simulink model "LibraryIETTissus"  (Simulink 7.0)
settings: Solver=ode45  StartTime=0.0  StopTime=10  RelTol=1e-3
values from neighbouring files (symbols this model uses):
  b = S/Sm    (= 0.1)    [Constantes.m]    (also in ConstantesBck.m)
  beta = 0.95    [Constantes.m]    (also in ResCourV1.m = 1; ResCrV1.m = 1; ResEnerV1.m = 1; ConstantesBck.m)
  C = 1    [Constantes.m]    (also in ConstantesBck.m)
  Cdl = 603E-9    (= 6.03e-07)    [Constantes.m]    (also in ResCourV1.m = 7.313e-07; ResCrV1.m = 7.313e-07; ResEnerV1.m = 7.313e-07; ConstantesBck.m)
  Cmem = 1E-6*Sm*(1-b)    (= 2.826e-08)    [Constantes.m]    (also in ConstantesBck.m = 3.14e-11; ImpedanceZtissus.m = 4e-08; Ztissus.m = 4e-08; CalculCharge.m = 1)
  Fact = 10^2    (= 100)    [Constantes.m]    (also in ConstantesBck.m)
  gk = 36    [Constantes.m]    (also in ConstantesBck.m; sim_hh.m)
  gl = 0.3    [Constantes.m]    (also in ConstantesBck.m; sim_hh.m)
  gna = 120    [Constantes.m]    (also in ConstantesBck.m; sim_hh.m)
  h0 = 0.5961    [Constantes.m]    (also in ConstantesBck.m)
  m0 = 0.0529    [Constantes.m]    (also in ConstantesBck.m)
  mK = 0    [Constantes.m]    (also in ConstantesBck.m)
  mL = 0    [Constantes.m]    (also in ConstantesBck.m)
  mNa = 0    [Constantes.m]    (also in ConstantesBck.m)
  n0 = 0.3177    [Constantes.m]    (also in ConstantesBck.m)
  rapportIE = 10    [Constantes.m]
  Rcan = 6.398E3*Sm*(1-b)    (= 180.80748)    [Constantes.m]    (also in ConstantesBck.m = 0.03454; ImpedanceZtissus.m = 44; Ztissus.m = 44)
  Rct = 185.6E3    (= 185600)    [Constantes.m]    (also in ResCourV1.m = 605200; ResCrV1.m = 605200; ResEnerV1.m = 605200; ConstantesBck.m)
  Rext = 2.9E3    (= 2900)    [Constantes.m]    (also in ConstantesBck.m)
  Rint = 2.9E2    (= 290)    [Constantes.m]    (also in ConstantesBck.m = 400)
  sigma = 66466    [Constantes.m]    (also in ResCourV1.m = 68000; ResCrV1.m = 68000; ResEnerV1.m = 68000; ConstantesBck.m)
  Sm = 3.14e-2    (= 0.0314)    [Constantes.m]    (also in ConstantesBck.m = 0.000314)
  Vk = -82    [Constantes.m]    (also in ConstantesBck.m)
  Vl = -59    [Constantes.m]    (also in ConstantesBck.m)
  Vna = 45    [Constantes.m]    (also in ConstantesBck.m)
  Vr = -70    [Constantes.m]    (also in ConstantesBck.m)
undefined symbols (not defined in the file or in its folder): ln
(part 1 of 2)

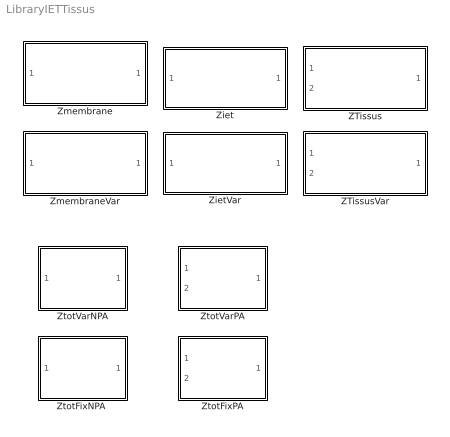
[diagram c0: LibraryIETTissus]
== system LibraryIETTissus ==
  ZTissus : Subsystem
  ZTissusVar : Subsystem
  Ziet : Subsystem
  ZietVar : Subsystem
  Zmembrane : Subsystem
  ZmembraneVar : Subsystem
  "ZtotFixNPA " : Subsystem
  ZtotFixPA : Subsystem
  ZtotVarNPA : Subsystem
  ZtotVarPA : Subsystem

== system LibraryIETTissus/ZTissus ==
  IStim : Inport  Orientation=left  OutDataType=sfix(16)  OutScaling=2^0
  Vref : Inport  Port=2  OutDataType=sfix(16)  OutScaling=2^0
  Constant : Constant  OutDataType=sfix(16)  OutScaling=2^0
  Contrôleur : Stateflow chart  Orientation=left
  Divide : Product  Inputs=*/  OutDataType=sfix(16)  OutScaling=2^-10
  Divide1 : Product  Inputs=*/  OutDataType=sfix(16)  OutScaling=2^-10
  Divide2 : Product  Inputs=*/  OutDataType=sfix(16)  OutScaling=2^-10
  Gain2 : Gain  Gain=Rext  ParameterDataType=sfix(16)  ParameterScaling=2^0  OutDataType=sfix(16)  OutScaling=2^0
  Sum1 : Sum  Inputs=|++  OutDataType=sfix(16)  OutScaling=2^0
  ZTissusInt : Subsystem
  Vout : Outport  Orientation=left  OutDataType=sfix(16)  OutScaling=2^0
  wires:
  Constant/1 -> Divide/1, Divide1/1, Divide2/1
  ZTissusInt/1(Vout) -> Divide/2
  Gain2/1 -> Divide1/2
  Divide/1 -> Sum1/1
  Divide1/1 -> Sum1/2
  Sum1/1 -> Divide2/2
  Vref/1 -> ZTissusInt/2(VRefIn)
  Divide2/1 -> Contrôleur/2(calc)
  Contrôleur/2(temp) -> ZTissusInt/1(InStim), Gain2/1
  IStim/1 -> Contrôleur/1(u)
  Contrôleur/1(y) -> Vout/1

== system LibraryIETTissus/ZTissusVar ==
  IStim : Inport  Orientation=left  OutDataType=sfix(16)  OutScaling=2^0
  Vref : Inport  Port=2  OutDataType=sfix(16)  OutScaling=2^0
  Constant : Constant  OutDataType=sfix(16)  OutScaling=2^0
  Contrôleur : Stateflow chart  Orientation=left
  Divide : Product  Inputs=*/  OutDataType=sfix(16)  OutScaling=2^-10
  Divide1 : Product  Inputs=*/  OutDataType=sfix(16)  OutScaling=2^-10
  Divide2 : Product  Inputs=*/  OutDataType=sfix(16)  OutScaling=2^-10
  Rext1 : Fcn  Expr=u*(1.6342*((abs(u)*1E6)^0.1267))*1E3
  Sum1 : Sum  Inputs=|++  OutDataType=sfix(16)  OutScaling=2^0
  ZTissusInt1 : Subsystem
  Vout : Outport  Orientation=left  OutDataType=sfix(16)  OutScaling=2^0
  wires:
  Constant/1 -> Divide/1, Divide1/1, Divide2/1
  ZTissusInt1/1(Vout) -> Divide/2
  Rext1/1 -> Divide1/2
  Divide/1 -> Sum1/1
  Divide1/1 -> Sum1/2
  Sum1/1 -> Divide2/2
  Vref/1 -> ZTissusInt1/2(VRefIn)
  Divide2/1 -> Contrôleur/2(calc)
  Contrôleur/2(temp) -> Rext1/1, ZTissusInt1/1(InStim)
  IStim/1 -> Contrôleur/1(u)
  Contrôleur/1(y) -> Vout/1

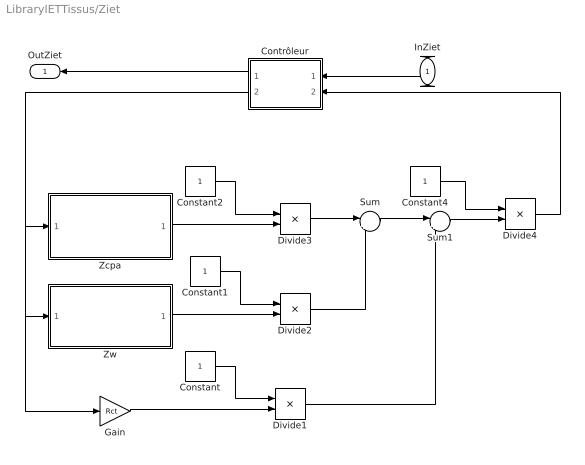
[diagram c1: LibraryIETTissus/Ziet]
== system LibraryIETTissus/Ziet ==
  InZiet : Inport  Orientation=left  OutDataType=sfix(16)  OutScaling=2^0
  Constant{,1..2,4} (4 alike) : Constant  OutDataType=sfix(16)  OutScaling=2^0
  Contrôleur : Stateflow chart  Orientation=left
  Divide{1..4} (4 alike) : Product  Inputs=*/  OutDataType=sfix(16)  OutScaling=2^-10
  Gain : Gain  Gain=Rct  ParameterDataType=sfix(16)  ParameterScaling=2^0  OutDataType=sfix(16)  OutScaling=2^0
  Sum : Sum  Inputs=|++  OutDataType=sfix(16)  OutScaling=2^0
  Sum1 : Sum  Inputs=|++  OutDataType=sfix(16)  OutScaling=2^0
  Zcpa : Subsystem
  Zw : Subsystem
  OutZiet : Outport  Orientation=left  OutDataType=sfix(16)  OutScaling=2^0
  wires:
  Constant/1 -> Divide1/1
  Constant1/1 -> Divide2/1
  Constant2/1 -> Divide3/1
  Zcpa/1(OutZcpa) -> Divide3/2
  Zw/1(OutZw) -> Divide2/2
  Divide3/1 -> Sum/1
  Constant4/1 -> Divide4/1
  Divide2/1 -> Sum/2
  Sum/1 -> Sum1/1
  Divide1/1 -> Sum1/2
  Sum1/1 -> Divide4/2
  Divide4/1 -> Contrôleur/2(calc)
  Gain/1 -> Divide1/2
  InZiet/1 -> Contrôleur/1(u)
  Contrôleur/1(y) -> OutZiet/1
  Contrôleur/2(temp) -> Zcpa/1(InZcpa), Zw/1(InZw), Gain/1

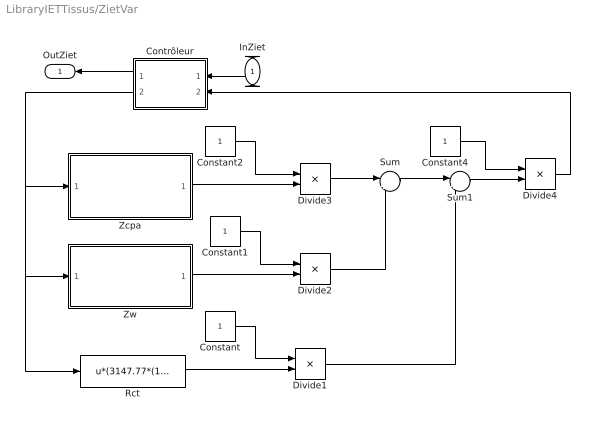
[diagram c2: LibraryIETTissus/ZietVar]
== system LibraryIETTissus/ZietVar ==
  InZiet : Inport  Orientation=left  OutDataType=sfix(16)  OutScaling=2^0
  Constant{,1..2,4} (4 alike) : Constant  OutDataType=sfix(16)  OutScaling=2^0
  Contrôleur : Stateflow chart  Orientation=left
  Divide{1..4} (4 alike) : Product  Inputs=*/  OutDataType=sfix(16)  OutScaling=2^-10
  Rct : Fcn  Expr=u*(3147.77*(1/((1E6*abs(u))^0.7199)))*1000
  Sum : Sum  Inputs=|++  OutDataType=sfix(16)  OutScaling=2^0
  Sum1 : Sum  Inputs=|++  OutDataType=sfix(16)  OutScaling=2^0
  Zcpa : Subsystem
  Zw : Subsystem
  OutZiet : Outport  Orientation=left  OutDataType=sfix(16)  OutScaling=2^0
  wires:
  Constant/1 -> Divide1/1
  Constant1/1 -> Divide2/1
  Constant2/1 -> Divide3/1
  Zcpa/1(OutZcpa) -> Divide3/2
  Zw/1(OutZw) -> Divide2/2
  Rct/1 -> Divide1/2
  Divide3/1 -> Sum/1
  Constant4/1 -> Divide4/1
  Divide2/1 -> Sum/2
  Sum/1 -> Sum1/1
  Divide1/1 -> Sum1/2
  Sum1/1 -> Divide4/2
  Contrôleur/2(temp) -> Rct/1, Zw/1(InZw), Zcpa/1(InZcpa)
  InZiet/1 -> Contrôleur/1(u)
  Contrôleur/1(y) -> OutZiet/1
  Divide4/1 -> Contrôleur/2(calc)

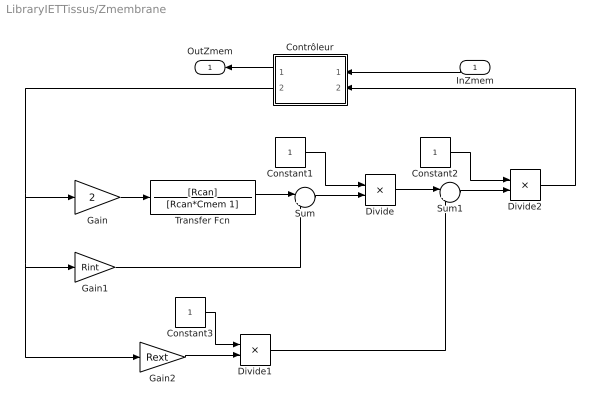
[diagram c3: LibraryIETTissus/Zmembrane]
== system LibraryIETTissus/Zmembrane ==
  InZmem : Inport  Orientation=left  OutDataType=sfix(16)  OutScaling=2^0
  Constant1 : Constant  OutDataType=sfix(16)  OutScaling=2^0
  Constant2 : Constant  OutDataType=sfix(16)  OutScaling=2^0
  Constant3 : Constant  OutDataType=sfix(16)  OutScaling=2^0
  Contrôleur : Stateflow chart  Orientation=left
  Divide : Product  Inputs=*/  OutDataType=sfix(16)  OutScaling=2^-10
  Divide1 : Product  Inputs=*/  OutDataType=sfix(16)  OutScaling=2^-10
  Divide2 : Product  Inputs=*/  OutDataType=sfix(16)  OutScaling=2^-10
  Gain : Gain  Gain=2  ParameterDataType=sfix(16)  ParameterScaling=2^0  OutDataType=sfix(16)  OutScaling=2^0
  Gain1 : Gain  Gain=Rint  ParameterDataType=sfix(16)  ParameterScaling=2^0  OutDataType=sfix(16)  OutScaling=2^0
  Gain2 : Gain  Gain=Rext  ParameterDataType=sfix(16)  ParameterScaling=2^0  OutDataType=sfix(16)  OutScaling=2^0
  Sum : Sum  Inputs=|++  OutDataType=sfix(16)  OutScaling=2^0
  Sum1 : Sum  Inputs=|++  OutDataType=sfix(16)  OutScaling=2^0
  Transfer Fcn : TransferFcn  Numerator=[Rcan]  Denominator=[Rcan*Cmem 1]
  OutZmem : Outport  Orientation=left  OutDataType=sfix(16)  OutScaling=2^0
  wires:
  Gain/1 -> Transfer Fcn/1
  Transfer Fcn/1 -> Sum/1
  Sum/1 -> Divide/2
  Gain2/1 -> Divide1/2
  Constant1/1 -> Divide/1
  Divide/1 -> Sum1/1
  Constant2/1 -> Divide2/1
  Sum1/1 -> Divide2/2
  Gain1/1 -> Sum/2
  Divide1/1 -> Sum1/2
  Divide2/1 -> Contrôleur/2(calc)
  Constant3/1 -> Divide1/1
  Contrôleur/2(temp) -> Gain2/1, Gain1/1, Gain/1
  InZmem/1 -> Contrôleur/1(u)
  Contrôleur/1(y) -> OutZmem/1

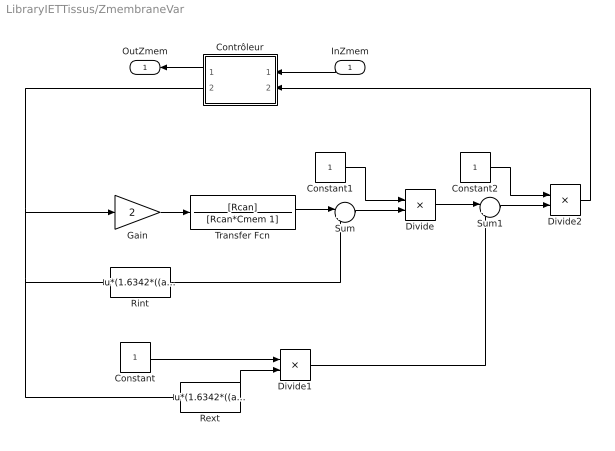
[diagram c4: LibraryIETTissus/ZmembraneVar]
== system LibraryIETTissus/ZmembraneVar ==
  InZmem : Inport  Orientation=left  OutDataType=sfix(16)  OutScaling=2^0
  Constant : Constant  OutDataType=sfix(16)  OutScaling=2^0
  Constant1 : Constant  OutDataType=sfix(16)  OutScaling=2^0
  Constant2 : Constant  OutDataType=sfix(16)  OutScaling=2^0
  Contrôleur : Stateflow chart  Orientation=left
  Divide : Product  Inputs=*/  OutDataType=sfix(16)  OutScaling=2^-10
  Divide1 : Product  Inputs=*/  OutDataType=sfix(16)  OutScaling=2^-10
  Divide2 : Product  Inputs=*/  OutDataType=sfix(16)  OutScaling=2^-10
  Gain : Gain  Gain=2  ParameterDataType=sfix(16)  ParameterScaling=2^0  OutDataType=sfix(16)  OutScaling=2^0
  Rext : Fcn  Expr=u*(1.6342*((abs(u)*1E6)^0.1267))*1E3
  Rint : Fcn  Expr=u*(1.6342*((abs(u)*1E6)^0.1267))*1E3/rapportIE
  Sum : Sum  Inputs=|++  OutDataType=sfix(16)  OutScaling=2^0
  Sum1 : Sum  Inputs=|++  OutDataType=sfix(16)  OutScaling=2^0
  Transfer Fcn : TransferFcn  Numerator=[Rcan]  Denominator=[Rcan*Cmem 1]
  OutZmem : Outport  Orientation=left  OutDataType=sfix(16)  OutScaling=2^0
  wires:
  Gain/1 -> Transfer Fcn/1
  Transfer Fcn/1 -> Sum/1
  Sum/1 -> Divide/2
  Rext/1 -> Divide1/2
  Constant1/1 -> Divide/1
  Constant/1 -> Divide1/1
  Divide/1 -> Sum1/1
  Constant2/1 -> Divide2/1
  Sum1/1 -> Divide2/2
  Rint/1 -> Sum/2
  Divide1/1 -> Sum1/2
  Contrôleur/2(temp) -> Rext/1, Rint/1, Gain/1
  Divide2/1 -> Contrôleur/2(calc)
  InZmem/1 -> Contrôleur/1(u)
  Contrôleur/1(y) -> OutZmem/1

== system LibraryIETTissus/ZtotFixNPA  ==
  InZtot : Inport  OutDataType=sfix(16)  OutScaling=2^0
  Gain : Gain  ParameterDataType=sfix(16)  ParameterScaling=2^0  OutDataType=sfix(16)  OutScaling=2^0
  Sum : Sum  Inputs=|++  OutDataType=sfix(16)  OutScaling=2^0
  Ziet : Subsystem
  Zmembrane : Subsystem
  OutZtot : Outport  OutDataType=sfix(16)  OutScaling=2^0
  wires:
  Ziet/1(OutZiet) -> Gain/1
  Zmembrane/1(OutZmem) -> Sum/1
  InZtot/1 -> Zmembrane/1(InZmem), Ziet/1(InZiet)
  Gain/1 -> Sum/2
  Sum/1 -> OutZtot/1

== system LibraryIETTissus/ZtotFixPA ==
  InZtot : Inport  OutDataType=sfix(16)  OutScaling=2^0
  InVref : Inport  Port=2  OutDataType=sfix(16)  OutScaling=2^0
  Gain : Gain  ParameterDataType=sfix(16)  ParameterScaling=2^0  OutDataType=sfix(16)  OutScaling=2^0
  Sum : Sum  Inputs=|++  OutDataType=sfix(16)  OutScaling=2^0
  ZTissus : Subsystem
  Ziet : Subsystem
  OutZtot : Outport  OutDataType=sfix(16)  OutScaling=2^0
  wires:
  ZTissus/1(Vout) -> Sum/2
  Ziet/1(OutZiet) -> Gain/1
  InZtot/1 -> Ziet/1(InZiet), ZTissus/1(IStim)
  Sum/1 -> OutZtot/1
  Gain/1 -> Sum/1
  InVref/1 -> ZTissus/2(Vref)

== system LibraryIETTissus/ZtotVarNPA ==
  InZtot : Inport  OutDataType=sfix(16)  OutScaling=2^0
  Gain : Gain  ParameterDataType=sfix(16)  ParameterScaling=2^0  OutDataType=sfix(16)  OutScaling=2^0
  Sum : Sum  Inputs=|++  OutDataType=sfix(16)  OutScaling=2^0
  ZietVar : Subsystem
  ZmembraneVar : Subsystem
  OutZtot : Outport  OutDataType=sfix(16)  OutScaling=2^0
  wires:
  ZietVar/1(OutZiet) -> Gain/1
  ZmembraneVar/1(OutZmem) -> Sum/1
  InZtot/1 -> ZmembraneVar/1(InZmem), ZietVar/1(InZiet)
  Gain/1 -> Sum/2
  Sum/1 -> OutZtot/1

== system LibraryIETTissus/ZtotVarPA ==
  InZtot : Inport  OutDataType=sfix(16)  OutScaling=2^0
  InVref : Inport  Port=2  OutDataType=sfix(16)  OutScaling=2^0
  Gain : Gain  ParameterDataType=sfix(16)  ParameterScaling=2^0  OutDataType=sfix(16)  OutScaling=2^0
  Sum : Sum  Inputs=|++  OutDataType=sfix(16)  OutScaling=2^0
  ZTissusVar : Subsystem
  ZietVar : Subsystem
  OutZtot : Outport  OutDataType=sfix(16)  OutScaling=2^0
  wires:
  ZietVar/1(OutZiet) -> Gain/1
  ZTissusVar/1(Vout) -> Sum/1
  InZtot/1 -> ZietVar/1(InZiet), ZTissusVar/1(IStim)
  Gain/1 -> Sum/2
  Sum/1 -> OutZtot/1
  InVref/1 -> ZTissusVar/2(Vref)

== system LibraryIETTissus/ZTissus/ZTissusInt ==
  InStim : Inport  Orientation=down  OutDataType=sfix(16)  OutScaling=2^0
  VRefIn : Inport  Port=2  OutDataType=sfix(16)  OutScaling=2^0
  Gain1 : Gain  Gain=Rint  ParameterDataType=sfix(16)  ParameterScaling=2^0  OutDataType=sfix(16)  OutScaling=2^0
  Gain2 : Gain  Gain=-1  ParameterDataType=sfix(16)  ParameterScaling=2^0  OutDataType=sfix(16)  OutScaling=2^0
  Gain3 : Gain  ParameterDataType=sfix(16)  ParameterScaling=2^0  OutDataType=sfix(16)  OutScaling=2^0
  Gain4 : Gain  Gain=-1  ParameterDataType=sfix(16)  ParameterScaling=2^0  OutDataType=sfix(16)  OutScaling=2^0
  Modele HH : Subsystem
  Modele HHRetour : Subsystem
  Sum1 : Sum  Inputs=|+++  OutDataType=sfix(16)  OutScaling=2^0
  Vout : Outport  OutDataType=sfix(16)  OutScaling=2^0
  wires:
  Modele HH/1(HHout) -> Gain3/1
  Modele HHRetour/1(HHout) -> Gain4/1
  Gain1/1 -> Sum1/2
  InStim/1 -> Gain1/1, Modele HHRetour/1(HHin), Gain2/1
  Sum1/1 -> Vout/1
  VRefIn/1 -> Modele HHRetour/2(VRefIn), Modele HH/2(VRefIn)
  Gain3/1 -> Sum1/1
  Gain4/1 -> Sum1/3
  Gain2/1 -> Modele HH/1(HHin)

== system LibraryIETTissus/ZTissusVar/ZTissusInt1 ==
  InStim : Inport  Orientation=down  OutDataType=sfix(16)  OutScaling=2^0
  VRefIn : Inport  Port=2  OutDataType=sfix(16)  OutScaling=2^0
  Gain2 : Gain  Gain=-1  ParameterDataType=sfix(16)  ParameterScaling=2^0  OutDataType=sfix(16)  OutScaling=2^0
  Gain3 : Gain  ParameterDataType=sfix(16)  ParameterScaling=2^0  OutDataType=sfix(16)  OutScaling=2^0
  Gain4 : Gain  Gain=-1  ParameterDataType=sfix(16)  ParameterScaling=2^0  OutDataType=sfix(16)  OutScaling=2^0
  Modele HH : Subsystem
  Modele HHRetour : Subsystem
  Rint : Fcn  Expr=u*(1.6342*((abs(u)*1E6)^0.1267))*1E3/rapportIE
  Sum1 : Sum  Inputs=|+++  OutDataType=sfix(16)  OutScaling=2^0
  Vout : Outport  OutDataType=sfix(16)  OutScaling=2^0
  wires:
  Modele HH/1(HHout) -> Gain3/1
  Modele HHRetour/1(HHout) -> Gain4/1
  Rint/1 -> Sum1/2
  InStim/1 -> Modele HHRetour/1(HHin), Rint/1, Gain2/1
  Sum1/1 -> Vout/1
  VRefIn/1 -> Modele HHRetour/2(VRefIn), Modele HH/2(VRefIn)
  Gain3/1 -> Sum1/1
  Gain4/1 -> Sum1/3
  Gain2/1 -> Modele HH/1(HHin)

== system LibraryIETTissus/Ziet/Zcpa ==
  InZcpa : Inport  OutDataType=sfix(16)  OutScaling=2^0
  Fcn : Fcn  Expr=u(1)^beta
  Transfer Fcn : TransferFcn  Denominator=[Cdl 0]
  OutZcpa : Outport  OutDataType=sfix(16)  OutScaling=2^0
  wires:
  Transfer Fcn/1 -> Fcn/1
  InZcpa/1 -> Transfer Fcn/1
  Fcn/1 -> OutZcpa/1

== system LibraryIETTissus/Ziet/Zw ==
  InZw : Inport  OutDataType=sfix(16)  OutScaling=2^0
  Gain : Gain  Gain=sigma  ParameterDataType=sfix(16)  ParameterScaling=2^0  OutDataType=sfix(16)  OutScaling=2^0
  Math Function : Math  Operator=sqrt  OutDataType=sfix(16)  OutScaling=2^0
  Transfer Fcn : TransferFcn  Numerator=[2]  Denominator=[1 0]
  OutZw : Outport  OutDataType=sfix(16)  OutScaling=2^0
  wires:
  Transfer Fcn/1 -> Math Function/1
  Math Function/1 -> Gain/1
  Gain/1 -> OutZw/1
  InZw/1 -> Transfer Fcn/1

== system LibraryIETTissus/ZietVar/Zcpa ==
  InZcpa : Inport  OutDataType=sfix(16)  OutScaling=2^0
  Cdl : Fcn  Expr=u*1E9/(918.15-80.854*ln(abs(u)*1E6))
  Fcn : Fcn  Expr=u(1)^beta
  Transfer Fcn : TransferFcn  Denominator=[1 0]
  OutZcpa : Outport  OutDataType=sfix(16)  OutScaling=2^0
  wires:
  Transfer Fcn/1 -> Fcn/1
  InZcpa/1 -> Cdl/1
  Fcn/1 -> OutZcpa/1
  Cdl/1 -> Transfer Fcn/1

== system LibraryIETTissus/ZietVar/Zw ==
  InZw : Inport  OutDataType=sfix(16)  OutScaling=2^0
  Math Function : Math  Operator=sqrt  OutDataType=sfix(16)  OutScaling=2^0
  Product : Product  OutDataType=sfix(16)  OutScaling=2^0
  Transfer Fcn : TransferFcn  Numerator=[2]  Denominator=[1 0]
  sigma : Fcn  Expr=(67202-0.0688*((1E6*abs(u))^2)-11.273*(1E6*abs(u)))
  OutZw : Outport  OutDataType=sfix(16)  OutScaling=2^0
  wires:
  Transfer Fcn/1 -> Math Function/1
  InZw/1 -> Transfer Fcn/1, sigma/1
  Math Function/1 -> Product/1
  sigma/1 -> Product/2
  Product/1 -> OutZw/1

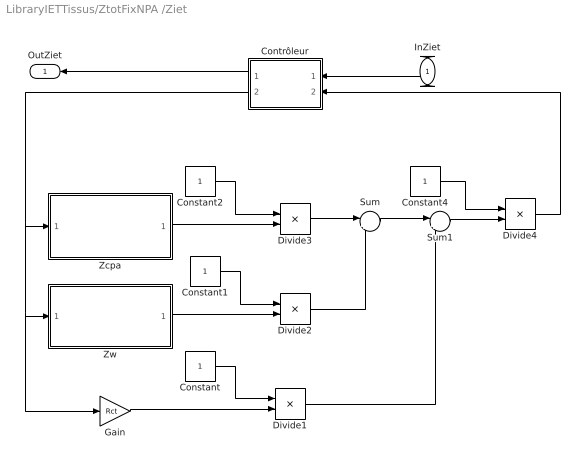
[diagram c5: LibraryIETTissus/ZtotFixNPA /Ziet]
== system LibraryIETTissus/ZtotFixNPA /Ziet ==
  InZiet : Inport  Orientation=left  OutDataType=sfix(16)  OutScaling=2^0
  Constant{,1..2,4} (4 alike) : Constant  OutDataType=sfix(16)  OutScaling=2^0
  Contrôleur : Stateflow chart  Orientation=left
  Divide{1..4} (4 alike) : Product  Inputs=*/  OutDataType=sfix(16)  OutScaling=2^-10
  Gain : Gain  Gain=Rct  ParameterDataType=sfix(16)  ParameterScaling=2^0  OutDataType=sfix(16)  OutScaling=2^0
  Sum : Sum  Inputs=|++  OutDataType=sfix(16)  OutScaling=2^0
  Sum1 : Sum  Inputs=|++  OutDataType=sfix(16)  OutScaling=2^0
  Zcpa : Subsystem
  Zw : Subsystem
  OutZiet : Outport  Orientation=left  OutDataType=sfix(16)  OutScaling=2^0
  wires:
  Constant/1 -> Divide1/1
  Constant1/1 -> Divide2/1
  Constant2/1 -> Divide3/1
  Zcpa/1(OutZcpa) -> Divide3/2
  Zw/1(OutZw) -> Divide2/2
  Divide3/1 -> Sum/1
  Constant4/1 -> Divide4/1
  Divide2/1 -> Sum/2
  Sum/1 -> Sum1/1
  Divide1/1 -> Sum1/2
  Sum1/1 -> Divide4/2
  Divide4/1 -> Contrôleur/2(calc)
  Gain/1 -> Divide1/2
  InZiet/1 -> Contrôleur/1(u)
  Contrôleur/1(y) -> OutZiet/1
  Contrôleur/2(temp) -> Zcpa/1(InZcpa), Zw/1(InZw), Gain/1

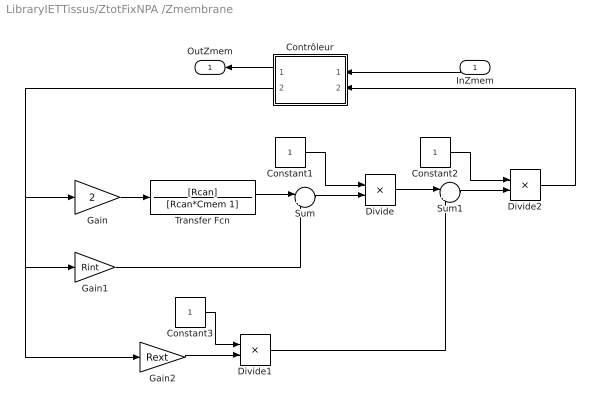
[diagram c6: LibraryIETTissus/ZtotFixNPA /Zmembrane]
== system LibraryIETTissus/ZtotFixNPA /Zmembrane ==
  InZmem : Inport  Orientation=left  OutDataType=sfix(16)  OutScaling=2^0
  Constant1 : Constant  OutDataType=sfix(16)  OutScaling=2^0
  Constant2 : Constant  OutDataType=sfix(16)  OutScaling=2^0
  Constant3 : Constant  OutDataType=sfix(16)  OutScaling=2^0
  Contrôleur : Stateflow chart  Orientation=left
  Divide : Product  Inputs=*/  OutDataType=sfix(16)  OutScaling=2^-10
  Divide1 : Product  Inputs=*/  OutDataType=sfix(16)  OutScaling=2^-10
  Divide2 : Product  Inputs=*/  OutDataType=sfix(16)  OutScaling=2^-10
  Gain : Gain  Gain=2  ParameterDataType=sfix(16)  ParameterScaling=2^0  OutDataType=sfix(16)  OutScaling=2^0
  Gain1 : Gain  Gain=Rint  ParameterDataType=sfix(16)  ParameterScaling=2^0  OutDataType=sfix(16)  OutScaling=2^0
  Gain2 : Gain  Gain=Rext  ParameterDataType=sfix(16)  ParameterScaling=2^0  OutDataType=sfix(16)  OutScaling=2^0
  Sum : Sum  Inputs=|++  OutDataType=sfix(16)  OutScaling=2^0
  Sum1 : Sum  Inputs=|++  OutDataType=sfix(16)  OutScaling=2^0
  Transfer Fcn : TransferFcn  Numerator=[Rcan]  Denominator=[Rcan*Cmem 1]
  OutZmem : Outport  Orientation=left  OutDataType=sfix(16)  OutScaling=2^0
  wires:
  Gain/1 -> Transfer Fcn/1
  Transfer Fcn/1 -> Sum/1
  Sum/1 -> Divide/2
  Gain2/1 -> Divide1/2
  Constant1/1 -> Divide/1
  Divide/1 -> Sum1/1
  Constant2/1 -> Divide2/1
  Sum1/1 -> Divide2/2
  Gain1/1 -> Sum/2
  Divide1/1 -> Sum1/2
  Divide2/1 -> Contrôleur/2(calc)
  Constant3/1 -> Divide1/1
  Contrôleur/2(temp) -> Gain2/1, Gain1/1, Gain/1
  InZmem/1 -> Contrôleur/1(u)
  Contrôleur/1(y) -> OutZmem/1

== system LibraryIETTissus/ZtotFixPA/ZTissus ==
  IStim : Inport  Orientation=left  OutDataType=sfix(16)  OutScaling=2^0
  Vref : Inport  Port=2  OutDataType=sfix(16)  OutScaling=2^0
  Constant : Constant  OutDataType=sfix(16)  OutScaling=2^0
  Contrôleur : Stateflow chart  Orientation=left
  Divide : Product  Inputs=*/  OutDataType=sfix(16)  OutScaling=2^-10
  Divide1 : Product  Inputs=*/  OutDataType=sfix(16)  OutScaling=2^-10
  Divide2 : Product  Inputs=*/  OutDataType=sfix(16)  OutScaling=2^-10
  Gain2 : Gain  Gain=Rext  ParameterDataType=sfix(16)  ParameterScaling=2^0  OutDataType=sfix(16)  OutScaling=2^0
  Sum1 : Sum  Inputs=|++  OutDataType=sfix(16)  OutScaling=2^0
  ZTissusInt : Subsystem
  Vout : Outport  Orientation=left  OutDataType=sfix(16)  OutScaling=2^0
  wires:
  Constant/1 -> Divide/1, Divide1/1, Divide2/1
  ZTissusInt/1(Vout) -> Divide/2
  Gain2/1 -> Divide1/2
  Divide/1 -> Sum1/1
  Divide1/1 -> Sum1/2
  Sum1/1 -> Divide2/2
  Vref/1 -> ZTissusInt/2(VRefIn)
  Divide2/1 -> Contrôleur/2(calc)
  Contrôleur/2(temp) -> ZTissusInt/1(InStim), Gain2/1
  IStim/1 -> Contrôleur/1(u)
  Contrôleur/1(y) -> Vout/1

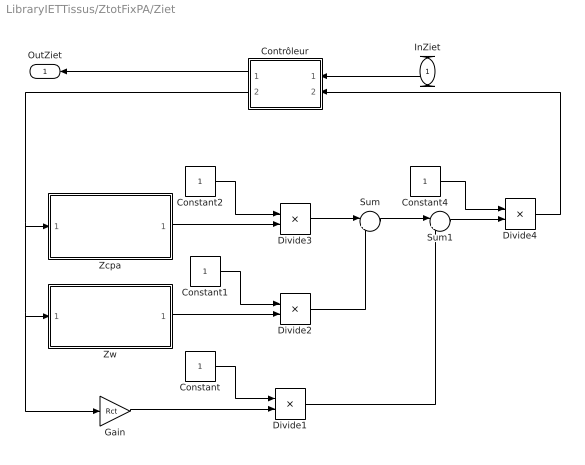
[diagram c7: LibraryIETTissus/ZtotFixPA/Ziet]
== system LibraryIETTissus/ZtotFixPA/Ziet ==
  InZiet : Inport  Orientation=left  OutDataType=sfix(16)  OutScaling=2^0
  Constant{,1..2,4} (4 alike) : Constant  OutDataType=sfix(16)  OutScaling=2^0
  Contrôleur : Stateflow chart  Orientation=left
  Divide{1..4} (4 alike) : Product  Inputs=*/  OutDataType=sfix(16)  OutScaling=2^-10
  Gain : Gain  Gain=Rct  ParameterDataType=sfix(16)  ParameterScaling=2^0  OutDataType=sfix(16)  OutScaling=2^0
  Sum : Sum  Inputs=|++  OutDataType=sfix(16)  OutScaling=2^0
  Sum1 : Sum  Inputs=|++  OutDataType=sfix(16)  OutScaling=2^0
  Zcpa : Subsystem
  Zw : Subsystem
  OutZiet : Outport  Orientation=left  OutDataType=sfix(16)  OutScaling=2^0
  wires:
  Constant/1 -> Divide1/1
  Constant1/1 -> Divide2/1
  Constant2/1 -> Divide3/1
  Zcpa/1(OutZcpa) -> Divide3/2
  Zw/1(OutZw) -> Divide2/2
  Divide3/1 -> Sum/1
  Constant4/1 -> Divide4/1
  Divide2/1 -> Sum/2
  Sum/1 -> Sum1/1
  Divide1/1 -> Sum1/2
  Sum1/1 -> Divide4/2
  Divide4/1 -> Contrôleur/2(calc)
  Gain/1 -> Divide1/2
  InZiet/1 -> Contrôleur/1(u)
  Contrôleur/1(y) -> OutZiet/1
  Contrôleur/2(temp) -> Zcpa/1(InZcpa), Zw/1(InZw), Gain/1

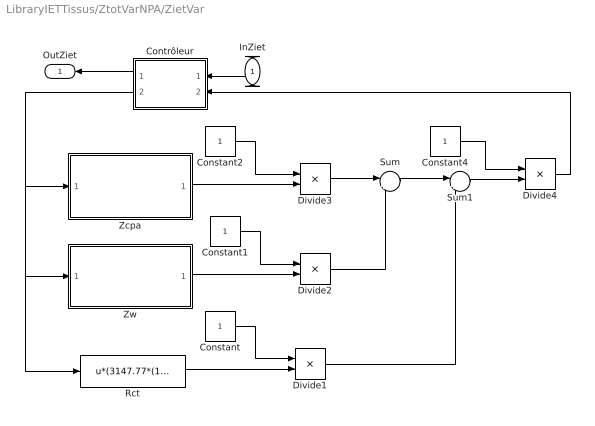
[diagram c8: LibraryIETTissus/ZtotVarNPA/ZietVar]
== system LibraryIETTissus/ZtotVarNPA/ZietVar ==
  InZiet : Inport  Orientation=left  OutDataType=sfix(16)  OutScaling=2^0
  Constant{,1..2,4} (4 alike) : Constant  OutDataType=sfix(16)  OutScaling=2^0
  Contrôleur : Stateflow chart  Orientation=left
  Divide{1..4} (4 alike) : Product  Inputs=*/  OutDataType=sfix(16)  OutScaling=2^-10
  Rct : Fcn  Expr=u*(3147.77*(1/((1E6*abs(u))^0.7199)))*1000
  Sum : Sum  Inputs=|++  OutDataType=sfix(16)  OutScaling=2^0
  Sum1 : Sum  Inputs=|++  OutDataType=sfix(16)  OutScaling=2^0
  Zcpa : Subsystem
  Zw : Subsystem
  OutZiet : Outport  Orientation=left  OutDataType=sfix(16)  OutScaling=2^0
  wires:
  Constant/1 -> Divide1/1
  Constant1/1 -> Divide2/1
  Constant2/1 -> Divide3/1
  Zcpa/1(OutZcpa) -> Divide3/2
  Zw/1(OutZw) -> Divide2/2
  Rct/1 -> Divide1/2
  Divide3/1 -> Sum/1
  Constant4/1 -> Divide4/1
  Divide2/1 -> Sum/2
  Sum/1 -> Sum1/1
  Divide1/1 -> Sum1/2
  Sum1/1 -> Divide4/2
  Contrôleur/2(temp) -> Rct/1, Zw/1(InZw), Zcpa/1(InZcpa)
  InZiet/1 -> Contrôleur/1(u)
  Contrôleur/1(y) -> OutZiet/1
  Divide4/1 -> Contrôleur/2(calc)

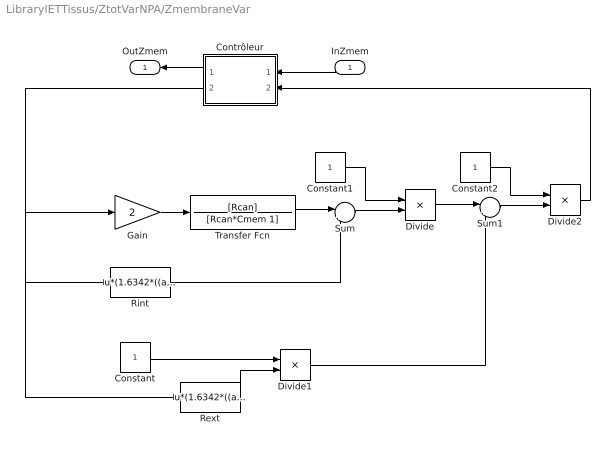
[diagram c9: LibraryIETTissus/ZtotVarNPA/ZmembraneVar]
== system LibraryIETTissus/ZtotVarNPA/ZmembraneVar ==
  InZmem : Inport  Orientation=left  OutDataType=sfix(16)  OutScaling=2^0
  Constant : Constant  OutDataType=sfix(16)  OutScaling=2^0
  Constant1 : Constant  OutDataType=sfix(16)  OutScaling=2^0
  Constant2 : Constant  OutDataType=sfix(16)  OutScaling=2^0
  Contrôleur : Stateflow chart  Orientation=left
  Divide : Product  Inputs=*/  OutDataType=sfix(16)  OutScaling=2^-10
  Divide1 : Product  Inputs=*/  OutDataType=sfix(16)  OutScaling=2^-10
  Divide2 : Product  Inputs=*/  OutDataType=sfix(16)  OutScaling=2^-10
  Gain : Gain  Gain=2  ParameterDataType=sfix(16)  ParameterScaling=2^0  OutDataType=sfix(16)  OutScaling=2^0
  Rext : Fcn  Expr=u*(1.6342*((abs(u)*1E6)^0.1267))*1E3
  Rint : Fcn  Expr=u*(1.6342*((abs(u)*1E6)^0.1267))*1E3/rapportIE
  Sum : Sum  Inputs=|++  OutDataType=sfix(16)  OutScaling=2^0
  Sum1 : Sum  Inputs=|++  OutDataType=sfix(16)  OutScaling=2^0
  Transfer Fcn : TransferFcn  Numerator=[Rcan]  Denominator=[Rcan*Cmem 1]
  OutZmem : Outport  Orientation=left  OutDataType=sfix(16)  OutScaling=2^0
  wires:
  Gain/1 -> Transfer Fcn/1
  Transfer Fcn/1 -> Sum/1
  Sum/1 -> Divide/2
  Rext/1 -> Divide1/2
  Constant1/1 -> Divide/1
  Constant/1 -> Divide1/1
  Divide/1 -> Sum1/1
  Constant2/1 -> Divide2/1
  Sum1/1 -> Divide2/2
  Rint/1 -> Sum/2
  Divide1/1 -> Sum1/2
  Contrôleur/2(temp) -> Rext/1, Rint/1, Gain/1
  Divide2/1 -> Contrôleur/2(calc)
  InZmem/1 -> Contrôleur/1(u)
  Contrôleur/1(y) -> OutZmem/1

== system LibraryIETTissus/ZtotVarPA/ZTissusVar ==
  IStim : Inport  Orientation=left  OutDataType=sfix(16)  OutScaling=2^0
  Vref : Inport  Port=2  OutDataType=sfix(16)  OutScaling=2^0
  Constant : Constant  OutDataType=sfix(16)  OutScaling=2^0
  Contrôleur : Stateflow chart  Orientation=left
  Divide : Product  Inputs=*/  OutDataType=sfix(16)  OutScaling=2^-10
  Divide1 : Product  Inputs=*/  OutDataType=sfix(16)  OutScaling=2^-10
  Divide2 : Product  Inputs=*/  OutDataType=sfix(16)  OutScaling=2^-10
  Rext1 : Fcn  Expr=u*(1.6342*((abs(u)*1E6)^0.1267))*1E3
  Sum1 : Sum  Inputs=|++  OutDataType=sfix(16)  OutScaling=2^0
  ZTissusInt1 : Subsystem
  Vout : Outport  Orientation=left  OutDataType=sfix(16)  OutScaling=2^0
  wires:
  Constant/1 -> Divide/1, Divide1/1, Divide2/1
  ZTissusInt1/1(Vout) -> Divide/2
  Rext1/1 -> Divide1/2
  Divide/1 -> Sum1/1
  Divide1/1 -> Sum1/2
  Sum1/1 -> Divide2/2
  Vref/1 -> ZTissusInt1/2(VRefIn)
  Divide2/1 -> Contrôleur/2(calc)
  Contrôleur/2(temp) -> Rext1/1, ZTissusInt1/1(InStim)
  IStim/1 -> Contrôleur/1(u)
  Contrôleur/1(y) -> Vout/1

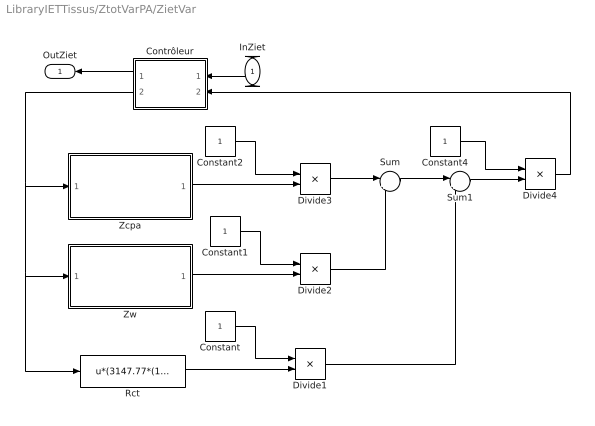
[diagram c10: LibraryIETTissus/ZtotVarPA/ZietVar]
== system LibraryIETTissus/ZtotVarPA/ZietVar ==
  InZiet : Inport  Orientation=left  OutDataType=sfix(16)  OutScaling=2^0
  Constant{,1..2,4} (4 alike) : Constant  OutDataType=sfix(16)  OutScaling=2^0
  Contrôleur : Stateflow chart  Orientation=left
  Divide{1..4} (4 alike) : Product  Inputs=*/  OutDataType=sfix(16)  OutScaling=2^-10
  Rct : Fcn  Expr=u*(3147.77*(1/((1E6*abs(u))^0.7199)))*1000
  Sum : Sum  Inputs=|++  OutDataType=sfix(16)  OutScaling=2^0
  Sum1 : Sum  Inputs=|++  OutDataType=sfix(16)  OutScaling=2^0
  Zcpa : Subsystem
  Zw : Subsystem
  OutZiet : Outport  Orientation=left  OutDataType=sfix(16)  OutScaling=2^0
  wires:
  Constant/1 -> Divide1/1
  Constant1/1 -> Divide2/1
  Constant2/1 -> Divide3/1
  Zcpa/1(OutZcpa) -> Divide3/2
  Zw/1(OutZw) -> Divide2/2
  Rct/1 -> Divide1/2
  Divide3/1 -> Sum/1
  Constant4/1 -> Divide4/1
  Divide2/1 -> Sum/2
  Sum/1 -> Sum1/1
  Divide1/1 -> Sum1/2
  Sum1/1 -> Divide4/2
  Contrôleur/2(temp) -> Rct/1, Zw/1(InZw), Zcpa/1(InZcpa)
  InZiet/1 -> Contrôleur/1(u)
  Contrôleur/1(y) -> OutZiet/1
  Divide4/1 -> Contrôleur/2(calc)

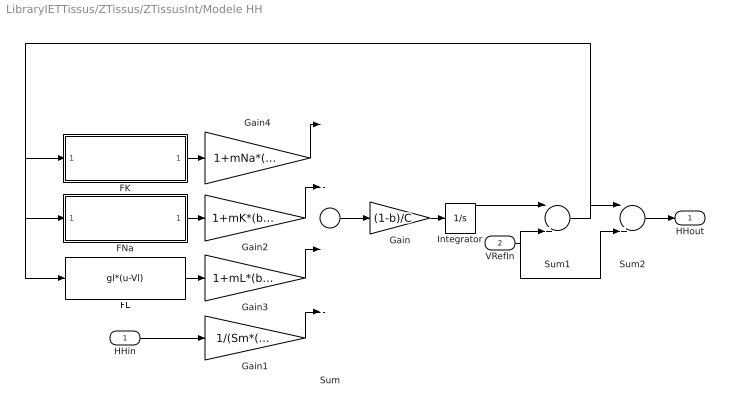
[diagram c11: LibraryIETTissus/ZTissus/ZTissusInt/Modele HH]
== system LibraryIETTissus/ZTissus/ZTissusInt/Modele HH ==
  HHin : Inport  OutDataType=sfix(16)  OutScaling=2^0
  VRefIn : Inport  Port=2  OutDataType=sfix(16)  OutScaling=2^0
  FK : Subsystem
  FL : Fcn  Expr=gl*(u-Vl)
  FNa : Subsystem
  Gain : Gain  Gain=(1-b)/C  ParameterDataType=sfix(16)  ParameterScaling=2^0  OutDataType=sfix(16)  OutScaling=2^0
  Gain1 : Gain  Gain=1/(Sm*(1-b))  ParameterDataType=sfix(16)  ParameterScaling=2^0  OutDataType=sfix(16)  OutScaling=2^0
  Gain2 : Gain  Gain=1+mK*(b/(1-b))  ParameterDataType=sfix(16)  ParameterScaling=2^0  OutDataType=sfix(16)  OutScaling=2^0
  Gain3 : Gain  Gain=1+mL*(b/(1-b))  ParameterDataType=sfix(16)  ParameterScaling=2^0  OutDataType=sfix(16)  OutScaling=2^0
  Gain4 : Gain  Gain=1+mNa*(b/(1-b))  ParameterDataType=sfix(16)  ParameterScaling=2^0  OutDataType=sfix(16)  OutScaling=2^0
  Integrator : Integrator  InitialCondition=Vr
  Sum : Sum  Inputs=|---+  OutDataType=sfix(16)  OutScaling=2^0
  Sum1 : Sum  Inputs=|++  OutDataType=sfix(16)  OutScaling=2^0
  Sum2 : Sum  Inputs=|+-  OutDataType=sfix(16)  OutScaling=2^0
  HHout : Outport  OutDataType=sfix(16)  OutScaling=2^0
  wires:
  Sum/1 -> Gain/1
  Gain/1 -> Integrator/1
  FK/1(FKout) -> Gain4/1
  FNa/1(FNaOut) -> Gain2/1
  FL/1 -> Gain3/1
  HHin/1 -> Gain1/1
  Integrator/1 -> Sum1/1
  Sum1/1 -> FNa/1(FNaIn), FL/1, FK/1(FKIn), Sum2/1
  VRefIn/1 -> Sum1/2, Sum2/2
  Gain1/1 -> Sum/4
  Gain4/1 -> Sum/1
  Gain2/1 -> Sum/2
  Gain3/1 -> Sum/3
  Sum2/1 -> HHout/1

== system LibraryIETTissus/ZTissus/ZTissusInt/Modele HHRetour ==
  HHin : Inport  OutDataType=sfix(16)  OutScaling=2^0
  VRefIn : Inport  Port=2  OutDataType=sfix(16)  OutScaling=2^0
  FK : Subsystem
  FL : Fcn  Expr=gl*(u-Vl)
  FNa : Subsystem
  Gain : Gain  Gain=(1-b)/C  ParameterDataType=sfix(16)  ParameterScaling=2^0  OutDataType=sfix(16)  OutScaling=2^0
  Gain1 : Gain  Gain=1/(Sm*(1-b))  ParameterDataType=sfix(16)  ParameterScaling=2^0  OutDataType=sfix(16)  OutScaling=2^0
  Gain2 : Gain  Gain=1+mK*(b/(1-b))  ParameterDataType=sfix(16)  ParameterScaling=2^0  OutDataType=sfix(16)  OutScaling=2^0
  Gain3 : Gain  Gain=1+mL*(b/(1-b))  ParameterDataType=sfix(16)  ParameterScaling=2^0  OutDataType=sfix(16)  OutScaling=2^0
  Gain4 : Gain  Gain=1+mNa*(b/(1-b))  ParameterDataType=sfix(16)  ParameterScaling=2^0  OutDataType=sfix(16)  OutScaling=2^0
  Integrator : Integrator  InitialCondition=Vr
  Sum : Sum  Inputs=|---+  OutDataType=sfix(16)  OutScaling=2^0
  Sum1 : Sum  Inputs=|++  OutDataType=sfix(16)  OutScaling=2^0
  Sum2 : Sum  Inputs=|+-  OutDataType=sfix(16)  OutScaling=2^0
  HHout : Outport  OutDataType=sfix(16)  OutScaling=2^0
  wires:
  Sum/1 -> Gain/1
  Gain/1 -> Integrator/1
  FK/1(FKout) -> Gain4/1
  FNa/1(FNaOut) -> Gain2/1
  FL/1 -> Gain3/1
  HHin/1 -> Gain1/1
  Integrator/1 -> Sum1/1
  Sum1/1 -> FNa/1(FNaIn), FL/1, FK/1(FKIn), Sum2/1
  VRefIn/1 -> Sum1/2, Sum2/2
  Gain1/1 -> Sum/4
  Gain4/1 -> Sum/1
  Gain2/1 -> Sum/2
  Gain3/1 -> Sum/3
  Sum2/1 -> HHout/1

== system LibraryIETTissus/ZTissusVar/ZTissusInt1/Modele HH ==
  HHin : Inport  OutDataType=sfix(16)  OutScaling=2^0
  VRefIn : Inport  Port=2  OutDataType=sfix(16)  OutScaling=2^0
  FK : Subsystem
  FL : Fcn  Expr=gl*(u-Vl)
  FNa : Subsystem
  Gain : Gain  Gain=(1-b)/C  ParameterDataType=sfix(16)  ParameterScaling=2^0  OutDataType=sfix(16)  OutScaling=2^0
  Gain1 : Gain  Gain=1/(Sm*(1-b)*Fact)  ParameterDataType=sfix(16)  ParameterScaling=2^0  OutDataType=sfix(16)  OutScaling=2^0
  Gain2 : Gain  Gain=1+mK*(b/(1-b))  ParameterDataType=sfix(16)  ParameterScaling=2^0  OutDataType=sfix(16)  OutScaling=2^0
  Gain3 : Gain  Gain=1+mL*(b/(1-b))  ParameterDataType=sfix(16)  ParameterScaling=2^0  OutDataType=sfix(16)  OutScaling=2^0
  Gain4 : Gain  Gain=1+mNa*(b/(1-b))  ParameterDataType=sfix(16)  ParameterScaling=2^0  OutDataType=sfix(16)  OutScaling=2^0
  Integrator : Integrator  InitialCondition=Vr
  Sum : Sum  Inputs=|---+  OutDataType=sfix(16)  OutScaling=2^0
  Sum1 : Sum  Inputs=|++  OutDataType=sfix(16)  OutScaling=2^0
  Sum2 : Sum  Inputs=|+-  OutDataType=sfix(16)  OutScaling=2^0
  HHout : Outport  OutDataType=sfix(16)  OutScaling=2^0
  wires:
  Sum/1 -> Gain/1
  Gain/1 -> Integrator/1
  FK/1(FKout) -> Gain4/1
  FNa/1(FNaOut) -> Gain2/1
  FL/1 -> Gain3/1
  HHin/1 -> Gain1/1
  Integrator/1 -> Sum1/1
  Sum1/1 -> FNa/1(FNaIn), FL/1, FK/1(FKIn), Sum2/1
  VRefIn/1 -> Sum1/2, Sum2/2
  Gain1/1 -> Sum/4
  Gain4/1 -> Sum/1
  Gain2/1 -> Sum/2
  Gain3/1 -> Sum/3
  Sum2/1 -> HHout/1

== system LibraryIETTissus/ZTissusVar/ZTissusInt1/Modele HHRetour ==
  HHin : Inport  OutDataType=sfix(16)  OutScaling=2^0
  VRefIn : Inport  Port=2  OutDataType=sfix(16)  OutScaling=2^0
  FK : Subsystem
  FL : Fcn  Expr=gl*(u-Vl)
  FNa : Subsystem
  Gain : Gain  Gain=(1-b)/C  ParameterDataType=sfix(16)  ParameterScaling=2^0  OutDataType=sfix(16)  OutScaling=2^0
  Gain1 : Gain  Gain=1/(Sm*(1-b)*Fact)  ParameterDataType=sfix(16)  ParameterScaling=2^0  OutDataType=sfix(16)  OutScaling=2^0
  Gain2 : Gain  Gain=1+mK*(b/(1-b))  ParameterDataType=sfix(16)  ParameterScaling=2^0  OutDataType=sfix(16)  OutScaling=2^0
  Gain3 : Gain  Gain=1+mL*(b/(1-b))  ParameterDataType=sfix(16)  ParameterScaling=2^0  OutDataType=sfix(16)  OutScaling=2^0
  Gain4 : Gain  Gain=1+mNa*(b/(1-b))  ParameterDataType=sfix(16)  ParameterScaling=2^0  OutDataType=sfix(16)  OutScaling=2^0
  Integrator : Integrator  InitialCondition=Vr
  Sum : Sum  Inputs=|---+  OutDataType=sfix(16)  OutScaling=2^0
  Sum1 : Sum  Inputs=|++  OutDataType=sfix(16)  OutScaling=2^0
  Sum2 : Sum  Inputs=|+-  OutDataType=sfix(16)  OutScaling=2^0
  HHout : Outport  OutDataType=sfix(16)  OutScaling=2^0
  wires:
  Sum/1 -> Gain/1
  Gain/1 -> Integrator/1
  FK/1(FKout) -> Gain4/1
  FNa/1(FNaOut) -> Gain2/1
  FL/1 -> Gain3/1
  HHin/1 -> Gain1/1
  Integrator/1 -> Sum1/1
  Sum1/1 -> FNa/1(FNaIn), FL/1, FK/1(FKIn), Sum2/1
  VRefIn/1 -> Sum1/2, Sum2/2
  Gain1/1 -> Sum/4
  Gain4/1 -> Sum/1
  Gain2/1 -> Sum/2
  Gain3/1 -> Sum/3
  Sum2/1 -> HHout/1

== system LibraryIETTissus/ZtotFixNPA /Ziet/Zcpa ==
  InZcpa : Inport  OutDataType=sfix(16)  OutScaling=2^0
  Fcn : Fcn  Expr=u^beta
  Transfer Fcn : TransferFcn  Denominator=[Cdl 0]
  OutZcpa : Outport  OutDataType=sfix(16)  OutScaling=2^0
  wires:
  Transfer Fcn/1 -> Fcn/1
  InZcpa/1 -> Transfer Fcn/1
  Fcn/1 -> OutZcpa/1

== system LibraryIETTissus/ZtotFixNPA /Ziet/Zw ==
  InZw : Inport  OutDataType=sfix(16)  OutScaling=2^0
  Gain : Gain  Gain=sigma  ParameterDataType=sfix(16)  ParameterScaling=2^0  OutDataType=sfix(16)  OutScaling=2^0
  Math Function : Math  Operator=sqrt  OutDataType=sfix(16)  OutScaling=2^0
  Transfer Fcn : TransferFcn  Numerator=[2]  Denominator=[1 0]
  OutZw : Outport  OutDataType=sfix(16)  OutScaling=2^0
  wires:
  Transfer Fcn/1 -> Math Function/1
  Math Function/1 -> Gain/1
  Gain/1 -> OutZw/1
  InZw/1 -> Transfer Fcn/1

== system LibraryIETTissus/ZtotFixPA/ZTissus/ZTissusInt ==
  InStim : Inport  Orientation=down  OutDataType=sfix(16)  OutScaling=2^0
  VRefIn : Inport  Port=2  OutDataType=sfix(16)  OutScaling=2^0
  Gain1 : Gain  Gain=Rint  ParameterDataType=sfix(16)  ParameterScaling=2^0  OutDataType=sfix(16)  OutScaling=2^0
  Gain2 : Gain  Gain=-1  ParameterDataType=sfix(16)  ParameterScaling=2^0  OutDataType=sfix(16)  OutScaling=2^0
  Gain3 : Gain  ParameterDataType=sfix(16)  ParameterScaling=2^0  OutDataType=sfix(16)  OutScaling=2^0
  Gain4 : Gain  Gain=-1  ParameterDataType=sfix(16)  ParameterScaling=2^0  OutDataType=sfix(16)  OutScaling=2^0
  Modele HH : Subsystem
  Modele HHRetour : Subsystem
  Sum1 : Sum  Inputs=|+++  OutDataType=sfix(16)  OutScaling=2^0
  Sum2 : Sum  Inputs=|+-  OutDataType=sfix(16)  OutScaling=2^0
  Vout : Outport  OutDataType=sfix(16)  OutScaling=2^0
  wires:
  Modele HH/1(HHout) -> Gain3/1
  Modele HHRetour/1(HHout) -> Gain4/1
  Gain1/1 -> Sum1/2
  InStim/1 -> Gain1/1, Modele HHRetour/1(HHin), Gain2/1
  Sum2/1 -> Modele HH/2(VRefIn)
  Sum1/1 -> Vout/1, Sum2/2
  VRefIn/1 -> Modele HHRetour/2(VRefIn), Sum2/1
  Gain3/1 -> Sum1/1
  Gain4/1 -> Sum1/3
  Gain2/1 -> Modele HH/1(HHin)

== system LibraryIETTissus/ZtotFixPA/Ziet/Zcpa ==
  InZcpa : Inport  OutDataType=sfix(16)  OutScaling=2^0
  Fcn : Fcn  Expr=u^beta
  Transfer Fcn : TransferFcn  Denominator=[Cdl 0]
  OutZcpa : Outport  OutDataType=sfix(16)  OutScaling=2^0
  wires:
  Transfer Fcn/1 -> Fcn/1
  InZcpa/1 -> Transfer Fcn/1
  Fcn/1 -> OutZcpa/1

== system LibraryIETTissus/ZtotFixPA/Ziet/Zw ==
  InZw : Inport  OutDataType=sfix(16)  OutScaling=2^0
  Gain : Gain  Gain=sigma  ParameterDataType=sfix(16)  ParameterScaling=2^0  OutDataType=sfix(16)  OutScaling=2^0
  Math Function : Math  Operator=sqrt  OutDataType=sfix(16)  OutScaling=2^0
  Transfer Fcn : TransferFcn  Numerator=[2]  Denominator=[1 0]
  OutZw : Outport  OutDataType=sfix(16)  OutScaling=2^0
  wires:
  Transfer Fcn/1 -> Math Function/1
  Math Function/1 -> Gain/1
  Gain/1 -> OutZw/1
  InZw/1 -> Transfer Fcn/1

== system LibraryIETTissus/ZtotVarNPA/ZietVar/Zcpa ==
  InZcpa : Inport  OutDataType=sfix(16)  OutScaling=2^0
  Cdl : Fcn  Expr=u*1E9/(918.15-80.854*ln(abs(u)*1E6))
  Fcn : Fcn  Expr=u^beta
  Transfer Fcn : TransferFcn  Denominator=[1 0]
  OutZcpa : Outport  OutDataType=sfix(16)  OutScaling=2^0
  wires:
  Transfer Fcn/1 -> Fcn/1
  InZcpa/1 -> Cdl/1
  Fcn/1 -> OutZcpa/1
  Cdl/1 -> Transfer Fcn/1

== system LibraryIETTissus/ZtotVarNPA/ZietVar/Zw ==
  InZw : Inport  OutDataType=sfix(16)  OutScaling=2^0
  Math Function : Math  Operator=sqrt  OutDataType=sfix(16)  OutScaling=2^0
  Product : Product  OutDataType=sfix(16)  OutScaling=2^0
  Transfer Fcn : TransferFcn  Numerator=[2]  Denominator=[1 0]
  sigma : Fcn  Expr=(67202-0.0688*((1E6*abs(u))^2)-11.273*(1E6*abs(u)))
  OutZw : Outport  OutDataType=sfix(16)  OutScaling=2^0
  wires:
  Transfer Fcn/1 -> Math Function/1
  InZw/1 -> Transfer Fcn/1, sigma/1
  Math Function/1 -> Product/1
  sigma/1 -> Product/2
  Product/1 -> OutZw/1

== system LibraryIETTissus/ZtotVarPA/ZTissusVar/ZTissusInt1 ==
  InStim : Inport  Orientation=down  OutDataType=sfix(16)  OutScaling=2^0
  VRefIn : Inport  Port=2  OutDataType=sfix(16)  OutScaling=2^0
  Gain2 : Gain  Gain=-1  ParameterDataType=sfix(16)  ParameterScaling=2^0  OutDataType=sfix(16)  OutScaling=2^0
  Gain3 : Gain  ParameterDataType=sfix(16)  ParameterScaling=2^0  OutDataType=sfix(16)  OutScaling=2^0
  Gain4 : Gain  Gain=-1  ParameterDataType=sfix(16)  ParameterScaling=2^0  OutDataType=sfix(16)  OutScaling=2^0
  Modele HH : Subsystem
  Modele HHRetour : Subsystem
  Rint : Fcn  Expr=u*(1.6342*((abs(u)*1E6)^0.1267))*1E3/rapportIE
  "Scope2 " : Scope
  Scope3 : Scope
  Sum1 : Sum  Inputs=|+++  OutDataType=sfix(16)  OutScaling=2^0
  Sum2 : Sum  Inputs=|+-  OutDataType=sfix(16)  OutScaling=2^0
  Vout : Outport  OutDataType=sfix(16)  OutScaling=2^0
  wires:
  Modele HH/1(HHout) -> Gain3/1
  Modele HHRetour/1(HHout) -> Gain4/1
  Rint/1 -> Sum1/2
  InStim/1 -> Modele HHRetour/1(HHin), Rint/1, Gain2/1
  Sum2/1 -> Modele HH/2(VRefIn)
  Sum1/1 -> Vout/1, Sum2/2
  VRefIn/1 -> Modele HHRetour/2(VRefIn), Sum2/1
  Gain3/1 -> Sum1/1, "Scope2 "/1
  Gain4/1 -> Sum1/3, Scope3/1
  Gain2/1 -> Modele HH/1(HHin)

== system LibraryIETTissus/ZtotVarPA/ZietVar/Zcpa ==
  InZcpa : Inport  OutDataType=sfix(16)  OutScaling=2^0
  Cdl : Fcn  Expr=u*1E9/(918.15-80.854*ln(abs(u)*1E6))
  Fcn : Fcn  Expr=u^beta
  Transfer Fcn : TransferFcn  Denominator=[1 0]
  OutZcpa : Outport  OutDataType=sfix(16)  OutScaling=2^0
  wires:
  Transfer Fcn/1 -> Fcn/1
  InZcpa/1 -> Cdl/1
  Fcn/1 -> OutZcpa/1
  Cdl/1 -> Transfer Fcn/1

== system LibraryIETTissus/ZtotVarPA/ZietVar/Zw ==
  InZw : Inport  OutDataType=sfix(16)  OutScaling=2^0
  Math Function : Math  Operator=sqrt  OutDataType=sfix(16)  OutScaling=2^0
  Product : Product  OutDataType=sfix(16)  OutScaling=2^0
  Transfer Fcn : TransferFcn  Numerator=[2]  Denominator=[1 0]
  sigma : Fcn  Expr=(67202-0.0688*((1E6*abs(u))^2)-11.273*(1E6*abs(u)))
  OutZw : Outport  OutDataType=sfix(16)  OutScaling=2^0
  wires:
  Transfer Fcn/1 -> Math Function/1
  InZw/1 -> Transfer Fcn/1, sigma/1
  Math Function/1 -> Product/1
  sigma/1 -> Product/2
  Product/1 -> OutZw/1

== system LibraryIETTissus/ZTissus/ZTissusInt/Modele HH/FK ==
  note: gkm
  note: (Vm-Vk0)
  FKIn : Inport  OutDataType=sfix(16)  OutScaling=2^0
  (Vm-Vk0) : Fcn  Expr=(u-Vk)
  Product : Product  OutDataType=sfix(16)  OutScaling=2^0
  n(Vm) : Subsystem
  n^4 : Fcn  Expr=gk*(u^4)
  FKout : Outport  OutDataType=sfix(16)  OutScaling=2^0  InitialOutput=0
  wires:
  n(Vm)/1(n) -> n^4/1
  (Vm-Vk0)/1 -> Product/2
  Product/1 -> FKout/1
  n^4/1 -> Product/1
  FKIn/1 -> n(Vm)/1(Vm), (Vm-Vk0)/1

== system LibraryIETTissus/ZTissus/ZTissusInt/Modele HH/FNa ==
  note: gNa*m^3
  note: m
  note: h
  note: gNam
  note: (Vm-VNa0)
  FNaIn : Inport  OutDataType=sfix(16)  OutScaling=2^0
  (Vm-VNa0) : Fcn  Expr=(u-Vna)
  Product : Product  OutDataType=sfix(16)  OutScaling=2^0
  Product1 : Product  OutDataType=sfix(16)  OutScaling=2^0
  gna*m^3 : Fcn  Expr=gna*u^3
  h(Vm) : Subsystem
  m(Vm) : Subsystem
  FNaOut : Outport  OutDataType=sfix(16)  OutScaling=2^0  InitialOutput=0
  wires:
  (Vm-VNa0)/1 -> Product1/2
  gna*m^3/1 -> Product/1
  Product1/1 -> FNaOut/1
  FNaIn/1 -> m(Vm)/1(Vm), h(Vm)/1(Vm), (Vm-VNa0)/1
  m(Vm)/1(n) -> gna*m^3/1
  h(Vm)/1(h) -> Product/2
  Product/1 -> Product1/1

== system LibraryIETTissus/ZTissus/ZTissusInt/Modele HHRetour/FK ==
  note: gkm
  note: (Vm-Vk0)
  FKIn : Inport  OutDataType=sfix(16)  OutScaling=2^0
  (Vm-Vk0) : Fcn  Expr=(u-Vk)
  Product : Product  OutDataType=sfix(16)  OutScaling=2^0
  n(Vm) : Subsystem
  n^4 : Fcn  Expr=gk*(u^4)
  FKout : Outport  OutDataType=sfix(16)  OutScaling=2^0  InitialOutput=0
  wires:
  n(Vm)/1(n) -> n^4/1
  (Vm-Vk0)/1 -> Product/2
  Product/1 -> FKout/1
  n^4/1 -> Product/1
  FKIn/1 -> n(Vm)/1(Vm), (Vm-Vk0)/1

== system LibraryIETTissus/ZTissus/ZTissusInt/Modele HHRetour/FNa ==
  note: gNa*m^3
  note: m
  note: h
  note: gNam
  note: (Vm-VNa0)
  FNaIn : Inport  OutDataType=sfix(16)  OutScaling=2^0
  (Vm-VNa0) : Fcn  Expr=(u-Vna)
  Product : Product  OutDataType=sfix(16)  OutScaling=2^0
  Product1 : Product  OutDataType=sfix(16)  OutScaling=2^0
  gna*m^3 : Fcn  Expr=gna*u^3
  h(Vm) : Subsystem
  m(Vm) : Subsystem
  FNaOut : Outport  OutDataType=sfix(16)  OutScaling=2^0  InitialOutput=0
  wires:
  (Vm-VNa0)/1 -> Product1/2
  gna*m^3/1 -> Product/1
  Product1/1 -> FNaOut/1
  FNaIn/1 -> m(Vm)/1(Vm), h(Vm)/1(Vm), (Vm-VNa0)/1
  m(Vm)/1(n) -> gna*m^3/1
  h(Vm)/1(h) -> Product/2
  Product/1 -> Product1/1

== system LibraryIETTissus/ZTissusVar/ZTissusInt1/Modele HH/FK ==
  note: gkm
  note: (Vm-Vk0)
  FKIn : Inport  OutDataType=sfix(16)  OutScaling=2^0
  (Vm-Vk0) : Fcn  Expr=(u-Vk)
  Product : Product  OutDataType=sfix(16)  OutScaling=2^0
  n(Vm) : Subsystem
  n^4 : Fcn  Expr=gk*(u^4)
  FKout : Outport  OutDataType=sfix(16)  OutScaling=2^0  InitialOutput=0
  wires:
  n(Vm)/1(n) -> n^4/1
  (Vm-Vk0)/1 -> Product/2
  Product/1 -> FKout/1
  n^4/1 -> Product/1
  FKIn/1 -> n(Vm)/1(Vm), (Vm-Vk0)/1

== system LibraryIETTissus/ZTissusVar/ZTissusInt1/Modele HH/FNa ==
  note: gNa*m^3
  note: m
  note: h
  note: gNam
  note: (Vm-VNa0)
  FNaIn : Inport  OutDataType=sfix(16)  OutScaling=2^0
  (Vm-VNa0) : Fcn  Expr=(u-Vna)
  Product : Product  OutDataType=sfix(16)  OutScaling=2^0
  Product1 : Product  OutDataType=sfix(16)  OutScaling=2^0
  gna*m^3 : Fcn  Expr=gna*u^3
  h(Vm) : Subsystem
  m(Vm) : Subsystem
  FNaOut : Outport  OutDataType=sfix(16)  OutScaling=2^0  InitialOutput=0
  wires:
  (Vm-VNa0)/1 -> Product1/2
  gna*m^3/1 -> Product/1
  Product1/1 -> FNaOut/1
  FNaIn/1 -> m(Vm)/1(Vm), h(Vm)/1(Vm), (Vm-VNa0)/1
  m(Vm)/1(n) -> gna*m^3/1
  h(Vm)/1(h) -> Product/2
  Product/1 -> Product1/1

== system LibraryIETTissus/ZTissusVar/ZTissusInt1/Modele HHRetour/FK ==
  note: gkm
  note: (Vm-Vk0)
  FKIn : Inport  OutDataType=sfix(16)  OutScaling=2^0
  (Vm-Vk0) : Fcn  Expr=(u-Vk)
  Product : Product  OutDataType=sfix(16)  OutScaling=2^0
  n(Vm) : Subsystem
  n^4 : Fcn  Expr=gk*(u^4)
  FKout : Outport  OutDataType=sfix(16)  OutScaling=2^0  InitialOutput=0
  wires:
  n(Vm)/1(n) -> n^4/1
  (Vm-Vk0)/1 -> Product/2
  Product/1 -> FKout/1
  n^4/1 -> Product/1
  FKIn/1 -> n(Vm)/1(Vm), (Vm-Vk0)/1

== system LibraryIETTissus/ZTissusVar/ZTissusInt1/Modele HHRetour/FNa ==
  note: gNa*m^3
  note: m
  note: h
  note: gNam
  note: (Vm-VNa0)
  FNaIn : Inport  OutDataType=sfix(16)  OutScaling=2^0
  (Vm-VNa0) : Fcn  Expr=(u-Vna)
  Product : Product  OutDataType=sfix(16)  OutScaling=2^0
  Product1 : Product  OutDataType=sfix(16)  OutScaling=2^0
  gna*m^3 : Fcn  Expr=gna*u^3
  h(Vm) : Subsystem
  m(Vm) : Subsystem
  FNaOut : Outport  OutDataType=sfix(16)  OutScaling=2^0  InitialOutput=0
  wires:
  (Vm-VNa0)/1 -> Product1/2
  gna*m^3/1 -> Product/1
  Product1/1 -> FNaOut/1
  FNaIn/1 -> m(Vm)/1(Vm), h(Vm)/1(Vm), (Vm-VNa0)/1
  m(Vm)/1(n) -> gna*m^3/1
  h(Vm)/1(h) -> Product/2
  Product/1 -> Product1/1

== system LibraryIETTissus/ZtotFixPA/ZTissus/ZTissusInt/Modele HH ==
  HHin : Inport  OutDataType=sfix(16)  OutScaling=2^0
  VRefIn : Inport  Port=2  OutDataType=sfix(16)  OutScaling=2^0
  FK : Subsystem
  FL : Fcn  Expr=gl*(u-Vl)
  FNa : Subsystem
  Gain : Gain  Gain=(1-b)/C  ParameterDataType=sfix(16)  ParameterScaling=2^0  OutDataType=sfix(16)  OutScaling=2^0
  Gain1 : Gain  Gain=1/(Sm*(1-b))  ParameterDataType=sfix(16)  ParameterScaling=2^0  OutDataType=sfix(16)  OutScaling=2^0
  Gain2 : Gain  Gain=1+mK*(b/(1-b))  ParameterDataType=sfix(16)  ParameterScaling=2^0  OutDataType=sfix(16)  OutScaling=2^0
  Gain3 : Gain  Gain=1+mL*(b/(1-b))  ParameterDataType=sfix(16)  ParameterScaling=2^0  OutDataType=sfix(16)  OutScaling=2^0
  Gain4 : Gain  Gain=1+mNa*(b/(1-b))  ParameterDataType=sfix(16)  ParameterScaling=2^0  OutDataType=sfix(16)  OutScaling=2^0
  Integrator : Integrator  InitialCondition=Vr
  Sum : Sum  Inputs=|---+  OutDataType=sfix(16)  OutScaling=2^0
  Sum1 : Sum  Inputs=|++  OutDataType=sfix(16)  OutScaling=2^0
  HHout : Outport  OutDataType=sfix(16)  OutScaling=2^0
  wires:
  Sum/1 -> Gain/1
  Gain/1 -> Integrator/1
  FK/1(FKout) -> Gain4/1
  FNa/1(FNaOut) -> Gain2/1
  FL/1 -> Gain3/1
  HHin/1 -> Gain1/1
  Integrator/1 -> Sum1/1
  Sum1/1 -> HHout/1, FNa/1(FNaIn), FL/1, FK/1(FKIn)
  VRefIn/1 -> Sum1/2
  Gain1/1 -> Sum/4
  Gain4/1 -> Sum/1
  Gain2/1 -> Sum/2
  Gain3/1 -> Sum/3

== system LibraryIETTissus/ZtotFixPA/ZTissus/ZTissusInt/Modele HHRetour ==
  HHin : Inport  OutDataType=sfix(16)  OutScaling=2^0
  VRefIn : Inport  Port=2  OutDataType=sfix(16)  OutScaling=2^0
  FK : Subsystem
  FL : Fcn  Expr=gl*(u-Vl)
  FNa : Subsystem
  Gain : Gain  Gain=(1-b)/C  ParameterDataType=sfix(16)  ParameterScaling=2^0  OutDataType=sfix(16)  OutScaling=2^0
  Gain1 : Gain  Gain=1/(Sm*(1-b)*Fact)  ParameterDataType=sfix(16)  ParameterScaling=2^0  OutDataType=sfix(16)  OutScaling=2^0
  Gain2 : Gain  Gain=1+mK*(b/(1-b))  ParameterDataType=sfix(16)  ParameterScaling=2^0  OutDataType=sfix(16)  OutScaling=2^0
  Gain3 : Gain  Gain=1+mL*(b/(1-b))  ParameterDataType=sfix(16)  ParameterScaling=2^0  OutDataType=sfix(16)  OutScaling=2^0
  Gain4 : Gain  Gain=1+mNa*(b/(1-b))  ParameterDataType=sfix(16)  ParameterScaling=2^0  OutDataType=sfix(16)  OutScaling=2^0
  Integrator : Integrator  InitialCondition=Vr
  Sum : Sum  Inputs=|---+  OutDataType=sfix(16)  OutScaling=2^0
  Sum1 : Sum  Inputs=|++  OutDataType=sfix(16)  OutScaling=2^0
  Sum2 : Sum  Inputs=|+-  OutDataType=sfix(16)  OutScaling=2^0
  HHout : Outport  OutDataType=sfix(16)  OutScaling=2^0
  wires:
  Sum/1 -> Gain/1
  Gain/1 -> Integrator/1
  FK/1(FKout) -> Gain4/1
  FNa/1(FNaOut) -> Gain2/1
  FL/1 -> Gain3/1
  HHin/1 -> Gain1/1
  Integrator/1 -> Sum1/1
  Sum1/1 -> FNa/1(FNaIn), FL/1, FK/1(FKIn), Sum2/1
  VRefIn/1 -> Sum1/2, Sum2/2
  Gain1/1 -> Sum/4
  Gain4/1 -> Sum/1
  Gain2/1 -> Sum/2
  Gain3/1 -> Sum/3
  Sum2/1 -> HHout/1

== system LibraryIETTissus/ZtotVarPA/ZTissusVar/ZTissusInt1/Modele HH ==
  HHin : Inport  OutDataType=sfix(16)  OutScaling=2^0
  VRefIn : Inport  Port=2  OutDataType=sfix(16)  OutScaling=2^0
  FK : Subsystem
  FL : Fcn  Expr=gl*(u-Vl)
  FNa : Subsystem
  Gain : Gain  Gain=(1-b)/C  ParameterDataType=sfix(16)  ParameterScaling=2^0  OutDataType=sfix(16)  OutScaling=2^0
  Gain1 : Gain  Gain=1/(Sm*(1-b))  ParameterDataType=sfix(16)  ParameterScaling=2^0  OutDataType=sfix(16)  OutScaling=2^0
  Gain2 : Gain  Gain=1+mK*(b/(1-b))  ParameterDataType=sfix(16)  ParameterScaling=2^0  OutDataType=sfix(16)  OutScaling=2^0
  Gain3 : Gain  Gain=1+mL*(b/(1-b))  ParameterDataType=sfix(16)  ParameterScaling=2^0  OutDataType=sfix(16)  OutScaling=2^0
  Gain4 : Gain  Gain=1+mNa*(b/(1-b))  ParameterDataType=sfix(16)  ParameterScaling=2^0  OutDataType=sfix(16)  OutScaling=2^0
  Integrator : Integrator  InitialCondition=Vr
  Sum : Sum  Inputs=|---+  OutDataType=sfix(16)  OutScaling=2^0
  Sum1 : Sum  Inputs=|++  OutDataType=sfix(16)  OutScaling=2^0
  HHout : Outport  OutDataType=sfix(16)  OutScaling=2^0
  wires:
  Sum/1 -> Gain/1
  Gain/1 -> Integrator/1
  FK/1(FKout) -> Gain4/1
  FNa/1(FNaOut) -> Gain2/1
  FL/1 -> Gain3/1
  HHin/1 -> Gain1/1
  Integrator/1 -> Sum1/1
  Sum1/1 -> HHout/1, FNa/1(FNaIn), FL/1, FK/1(FKIn)
  VRefIn/1 -> Sum1/2
  Gain1/1 -> Sum/4
  Gain4/1 -> Sum/1
  Gain2/1 -> Sum/2
  Gain3/1 -> Sum/3

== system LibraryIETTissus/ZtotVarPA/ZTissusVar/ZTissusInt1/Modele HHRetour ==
  HHin : Inport  OutDataType=sfix(16)  OutScaling=2^0
  VRefIn : Inport  Port=2  OutDataType=sfix(16)  OutScaling=2^0
  FK : Subsystem
  FL : Fcn  Expr=gl*(u-Vl)
  FNa : Subsystem
  Gain : Gain  Gain=(1-b)/C  ParameterDataType=sfix(16)  ParameterScaling=2^0  OutDataType=sfix(16)  OutScaling=2^0
  Gain1 : Gain  Gain=1/(Sm*(1-b)*Fact)  ParameterDataType=sfix(16)  ParameterScaling=2^0  OutDataType=sfix(16)  OutScaling=2^0
  Gain2 : Gain  Gain=1+mK*(b/(1-b))  ParameterDataType=sfix(16)  ParameterScaling=2^0  OutDataType=sfix(16)  OutScaling=2^0
  Gain3 : Gain  Gain=1+mL*(b/(1-b))  ParameterDataType=sfix(16)  ParameterScaling=2^0  OutDataType=sfix(16)  OutScaling=2^0
  Gain4 : Gain  Gain=1+mNa*(b/(1-b))  ParameterDataType=sfix(16)  ParameterScaling=2^0  OutDataType=sfix(16)  OutScaling=2^0
  Integrator : Integrator  InitialCondition=Vr
  Sum : Sum  Inputs=|---+  OutDataType=sfix(16)  OutScaling=2^0
  Sum1 : Sum  Inputs=|++  OutDataType=sfix(16)  OutScaling=2^0
  Sum2 : Sum  Inputs=|+-  OutDataType=sfix(16)  OutScaling=2^0
  HHout : Outport  OutDataType=sfix(16)  OutScaling=2^0
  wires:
  Sum/1 -> Gain/1
  Gain/1 -> Integrator/1
  FK/1(FKout) -> Gain4/1
  FNa/1(FNaOut) -> Gain2/1
  FL/1 -> Gain3/1
  HHin/1 -> Gain1/1
  Integrator/1 -> Sum1/1
  Sum1/1 -> FNa/1(FNaIn), FL/1, FK/1(FKIn), Sum2/1
  VRefIn/1 -> Sum1/2, Sum2/2
  Gain1/1 -> Sum/4
  Gain4/1 -> Sum/1
  Gain2/1 -> Sum/2
  Gain3/1 -> Sum/3
  Sum2/1 -> HHout/1
